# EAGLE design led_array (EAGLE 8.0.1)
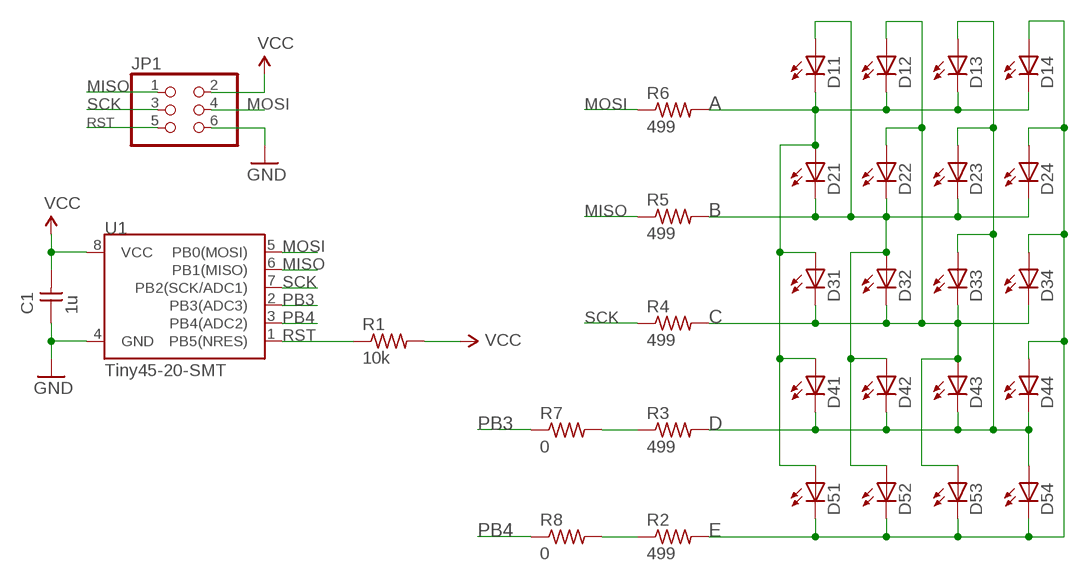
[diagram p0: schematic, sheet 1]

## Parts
C1  1u  CAP-UNPOLARIZEDFAB  [C1206FAB]
D11  LED  [LED1206]
D12  LED  [LED1206]
D13  LED  [LED1206]
D14  LED  [LED1206]
D21  LED  [LED1206]
D22  LED  [LED1206]
D23  LED  [LED1206]
D24  LED  [LED1206]
D31  LED  [LED1206]
D32  LED  [LED1206]
D33  LED  [LED1206]
D34  LED  [LED1206]
D41  LED  [LED1206]
D42  LED  [LED1206]
D43  LED  [LED1206]
D44  LED  [LED1206]
D51  LED  [LED1206]
D52  LED  [LED1206]
D53  LED  [LED1206]
D54  LED  [LED1206]
JP1  PINHD-2X3-SMD  [2X03SMD]
R1  10k  RES-US1206FAB  [R1206FAB]
R2  499  RES-US1206FAB  [R1206FAB]
R3  499  RES-US1206FAB  [R1206FAB]
R4  499  RES-US1206FAB  [R1206FAB]
R5  499  RES-US1206FAB  [R1206FAB]
R6  499  RES-US1206FAB  [R1206FAB]
R7  0  RES-US1206FAB  [R1206FAB]
R8  0  RES-US1206FAB  [R1206FAB]
U1  Tiny45-20-SMT  ATTINY45TINY45-20-SMT  [SO08-EIAJ]

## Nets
A: D11.2(C) D12.2(C) D13.2(C) D14.2(C) D21.1(A) D31.1(A) D41.1(A) D51.1(A) R6.2
B: D11.1(A) D21.2(C) D22.2(C) D23.2(C) D24.2(C) D32.1(A) D42.1(A) D52.1(A) R5.2
C: D12.1(A) D22.1(A) D31.2(C) D32.2(C) D33.2(C) D34.2(C) D43.1(A) D53.1(A) R4.2
D: D13.1(A) D23.1(A) D33.1(A) D41.2(C) D42.2(C) D43.2(C) D44.2(C) D54.1(A) R3.2
E: D14.1(A) D24.1(A) D34.1(A) D44.1(A) D51.2(C) D52.2(C) D53.2(C) D54.2(C) R2.2
GND: C1.1 JP1.6 U1.4(GND)
MISO: JP1.1 R5.1 U1.6(PB1(MISO))
MOSI: JP1.4 R6.1 U1.5(PB0(MOSI))
N$2: R3.1 R7.2
N$3: R2.1 R8.2
PB3: R7.1 U1.2(PB3(ADC3))
PB4: R8.1 U1.3(PB4(ADC2))
RST: JP1.5 R1.1 U1.1(PB5(NRES))
SCK: JP1.3 R4.1 U1.7(PB2(SCK/ADC1))
VCC: C1.2 JP1.2 R1.2 U1.8(VCC)

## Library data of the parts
C1 = 00fab:CAP-UNPOLARIZED
D11-D14 D21-D24 D31-D34 D41-D44 D51-D54 = 00fab:LED: LED
JP1 = 00fab:PINHD-2X3-SMD: PIN HEADER
R1-R8 = 00fab:RES-US: Resistor (US Symbol)
U1 = SparkFun-DigitalIC:ATTINY45: Atmel 8-pin 2/4/8kB flash uC; PROD_ID: IC-08922

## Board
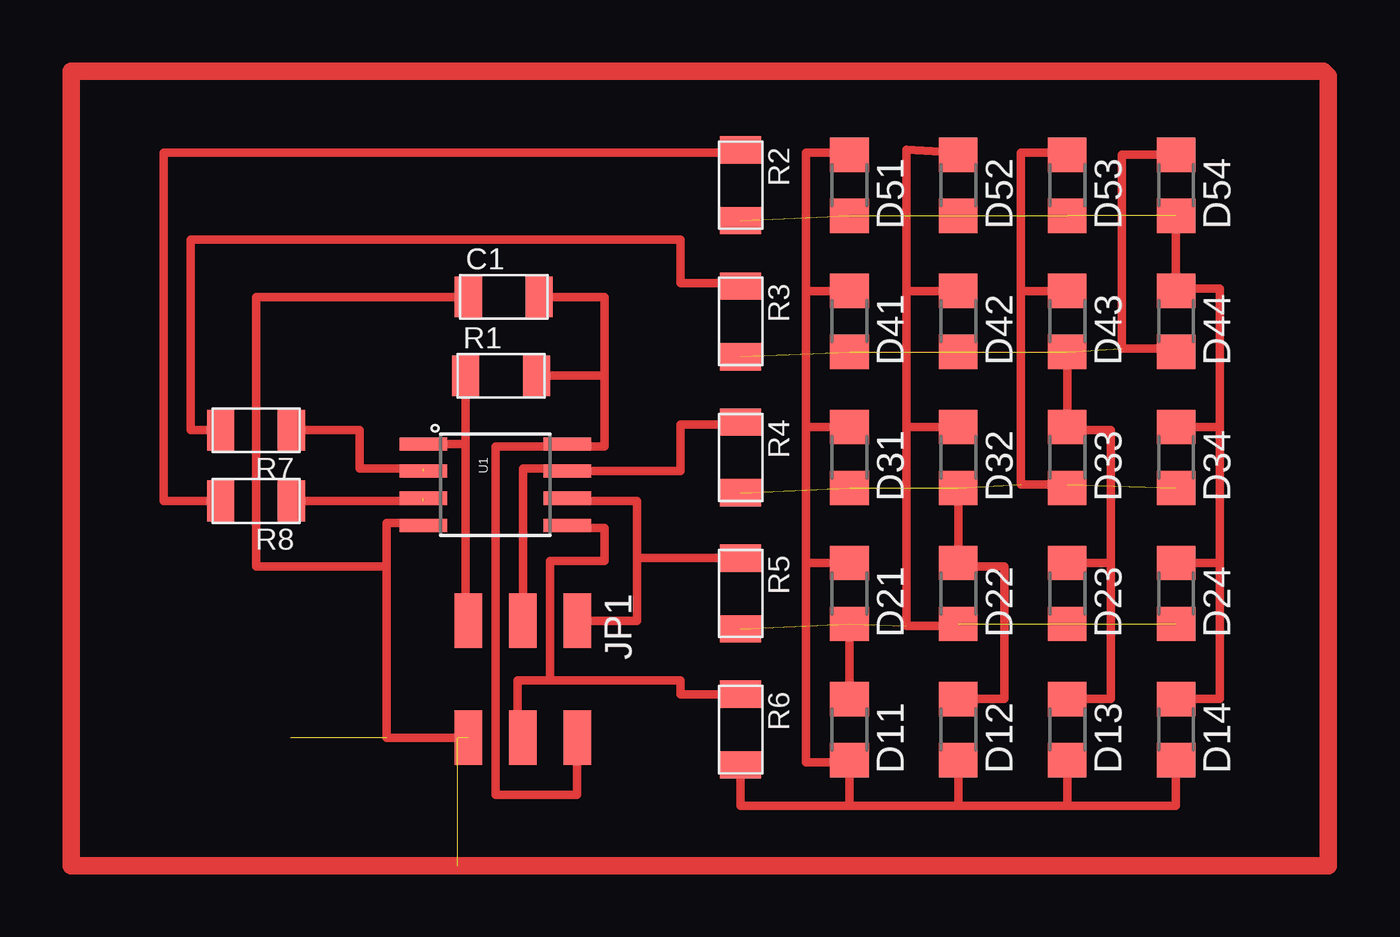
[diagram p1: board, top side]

No outline drawn. Coordinates in mm, seen from the top.
Copper layers (1*16): Top 0.035mm / dielectric 1.5mm / Bottom 0.035mm
Design rules "default *": minimum track width 10mil, minimum drill 24mil, track to track 10mil, track to pad 10mil, pad to pad 10mil, via to via 8mil, smd to smd 8mil, copper to edge 40mil, drill to drill 8mil, minimum pad ring 10mil, minimum via ring 8mil, stop-mask expansion 4mil, vias tented up to drill 0mil, thermal gap 10mil

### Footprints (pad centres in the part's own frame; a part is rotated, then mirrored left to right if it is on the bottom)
C1206FAB = smd 1.27 x 1.905: 1 -1.651,0; 2 1.651,0
LED1206 = smd 1.6 x 1.803: 1 -1.422,0; 2 1.422,0
2X03SMD = smd 2.54 x 1.27: 1 -2.54,2.54; 2 2.92,2.54; 3 -2.54,0; 4 2.92,0; 5 -2.54,-2.54; 6 2.92,-2.54
R1206FAB = smd 1.27 x 1.905: 1 -1.651,0; 2 1.651,0
SO08-EIAJ = smd 0.61 x 2.21: 1 -1.905,-3.378; 2 -0.635,-3.378; 3 0.635,-3.378; 4 1.905,-3.378; 5 1.905,3.353; 6 0.635,3.353; 7 -0.635,3.353; 8 -1.905,3.353

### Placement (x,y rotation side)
C1  19.94,31.62 0 top
D11  36.07,11.43 270 top
D12  41.15,11.43 270 top
D13  46.23,11.43 270 top
D14  51.31,11.43 270 top
D21  36.07,17.78 270 top
D22  41.15,17.78 270 top
D23  46.23,17.78 270 top
D24  51.31,17.78 270 top
D31  36.07,24.13 270 top
D32  41.15,24.13 270 top
D33  46.23,24.13 270 top
D34  51.31,24.13 270 top
D41  36.07,30.48 270 top
D42  41.15,30.48 270 top
D43  46.23,30.48 270 top
D44  51.31,30.48 270 top
D51  36.07,36.83 270 top
D52  41.15,36.83 270 top
D53  46.23,36.83 270 top
D54  51.31,36.83 270 top
JP1  20.83,13.97 270 top
R1  19.81,27.94 0 top
R2  30.99,36.83 270 top
R3  30.99,30.48 270 top
R4  30.99,24.13 270 top
R5  30.99,17.78 270 top
R6  30.99,11.43 270 top
R7  8.38,25.4 180 top
R8  8.38,22.1 180 top
U1  19.56,22.86 270 top

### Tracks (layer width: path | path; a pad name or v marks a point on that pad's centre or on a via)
A
  Top 0.406: 34.04,19.2 34.04,25.55 | 34.04,25.55 34.04,31.9 | 34.04,31.9 34.04,38.35 36.07,38.35 D51.1 | D41.1 34.04,31.9 | D31.1 34.04,25.55 | D21.1 34.04,19.2 | 34.04,19.2 34.04,9.91 36.07,9.91 D11.2 36.07,7.87 | R6.2 30.99,7.87 36.07,7.87 | 36.07,7.87 41.15,7.87 | 41.15,7.87 46.23,7.87 | 46.23,7.87 51.31,7.87 D14.2 | D12.2 41.15,7.87 | D13.2 46.23,7.87
B  (4 unrouted)
  Top 0.406: 38.73,25.55 38.73,31.9 | 38.73,31.9 38.73,38.48 41.15,38.35 D52.1 | D42.1 38.73,31.9 | D32.1 38.73,25.55 | 38.73,25.55 38.73,16.26 41.15,16.26 D22.2 | D21.2 D11.1
C  (4 unrouted)
  Top 0.406: 44.07,31.9 44.07,38.35 46.23,38.35 D53.1 | D43.1 44.07,31.9 | 44.07,31.9 44.07,22.86 46.23,22.86 D33.2 | D32.2 D22.1 41.15,19.05 43.31,19.05 43.31,12.85 D12.1
D  (4 unrouted)
  Top 0.406: D54.1 48.77,38.25 48.77,29.21 51.31,29.21 D44.2 | D43.2 D33.1 46.23,25.4 48.26,25.4 48.26,19.2 | D13.1 48.26,12.85 48.26,19.2 | D23.1 48.26,19.2
E  (4 unrouted)
  Top 0.406: D54.2 D44.1 51.31,32 53.34,32 53.34,25.55 | D34.1 53.34,25.55 | D14.1 53.34,12.85 53.34,19.2 | 53.34,19.2 53.34,25.55 | D24.1 53.34,19.2
GND  (3 unrouted)
  Top 0.406: JP1.6 14.48,11.05 14.48,19.05 | 14.48,19.05 14.48,21.08 16.18,21.08 U1.4 | C1.1 8.38,31.62 8.38,19.05 14.48,19.05
MISO
  Top 0.406: JP1.1 26.16,16.51 26.16,19.43 | 26.16,19.43 26.16,22.1 22.91,22.1 U1.6 | R5.1 26.16,19.43
MOSI
  Top 0.406: JP1.4 20.57,11.05 20.57,13.72 22.1,13.72 | 22.1,13.72 22.1,19.3 24.64,19.3 24.64,20.83 22.91,20.83 U1.5 | R6.1 28.19,13.08 28.19,13.72 22.1,13.72
N$2
  Top 0.406: R7.2 5.33,25.4 5.33,34.29 28.19,34.29 28.19,32.26 30.99,32.26 R3.1
N$3
  Top 0.406: R8.2 4.06,22.1 4.06,38.35 30.99,38.35 R2.1
N$5
  Top 0.813: -0.25,5.08 -0.25,42.16 58.17,42.16 58.42,41.91 58.42,5.08 -0.25,5.08
PB3  (1 unrouted)
  Top 0.406: R7.1 13.21,25.4 13.21,23.62 16.18,23.62
PB4  (1 unrouted)
  Top 0.406: R8.1 16.18,22.1
RST
  Top 0.406: R1.1 18.16,24.77 | 18.16,24.77 18.16,16.64 JP1.5 | U1.1 18.16,24.77
SCK
  Top 0.406: JP1.3 20.83,23.62 22.91,23.62 U1.7 28.19,23.5 28.19,25.65 30.99,25.65 R4.1
VCC
  Top 0.406: JP1.2 23.37,8.38 22.48,8.38 19.56,8.38 19.56,24.64 22.91,24.64 | R1.2 24.64,27.94 | 24.64,27.94 24.64,24.64 22.91,24.64 | 22.91,24.64 U1.8 | C1.2 24.64,31.62 24.64,27.94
